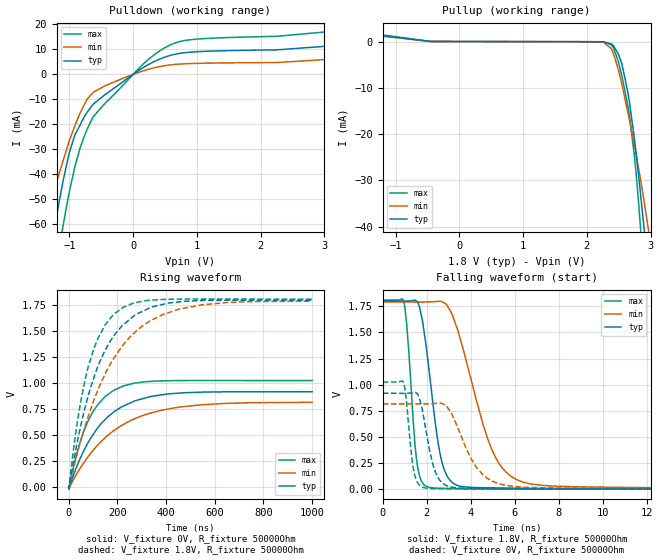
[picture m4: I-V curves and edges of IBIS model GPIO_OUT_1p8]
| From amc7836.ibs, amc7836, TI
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|   Model
[Model]   GPIO_OUT_1p8
Model_type   Output
Polarity   Non-Inverting
Vmeas = 0.9
Vref = 0
Cref = 1pF
Rref = 100000
|   typ   min   max
C_comp   2.855pF   2.622pF   2.914pF
[Voltage Range]   1.8   1.79   1.81
[Temperature Range]   27   125   -40
[Pullup Reference]   1.8   1.79   1.81
[Pulldown Reference]   0   0   0
[Power Clamp Reference]   1.8   1.79   1.81
[GND Clamp Reference]   0   0   0
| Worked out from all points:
|   slope of the pulldown table from 0 to 0.27 V, typ, clamps not added: 62.1 ohm
|   slope of the pullup table from 0 to 0.27 V, typ, clamps not added: 48 kohm
|   falling waveform, V_fixture 1.8V, R_fixture 50000Ohm: 20-80 % time 663ps typ, 1.47ns min, 359ps max; typ from 1.8 V to 0.004 V
|   rising waveform, V_fixture 0V, R_fixture 50000Ohm: 20-80 % time 161ns typ, 224ns min, 109ns max; typ from 0.002 V to 0.918 V
|   rising waveform, V_fixture 1.8V, R_fixture 50000Ohm: 20-80 % time 152ns typ, 207ns min, 104ns max; typ from 0.004 V to 1.8 V
|   falling waveform, V_fixture 0V, R_fixture 50000Ohm: 20-80 % time 539ps typ, 1.16ns min, 299ps max; typ from 0.919 V to 0.002 V
[Pulldown]
|   Voltage   I(typ)   I(min)   I(max)
-1.8V     -152.9mA   -105mA     -208.5mA
-1.422V   -90.58mA   -64.62mA   -123.9mA
-1.26V    -65.97mA   -48.83mA   -90.14mA
-1.199V   -56.75mA   -43.25mA   -77.47mA
-1.093V   -42.19mA   -34.3mA    -60.11mA
-995.4mV  -31.07mA   -26.33mA   -46.69mA
-833.4mV  -20.43mA   -15.7mA    -29.76mA
-644.4mV  -12.6mA    -7.83mA    -18mA
-444.6mV  -8.238mA   -4.696mA   -11.76mA
235.8mV   3.851mA    1.971mA    5.875mA
689.4mV   8.213mA    4.042mA    12.84mA
3.6V      12.34mA    6.871mA    18.33mA
[Pullup]
|   Voltage   I(typ)   I(min)   I(max)
-1.8V     2.219mA    2.026mA    2.51mA
-444.6mV  9.239uA    7.553uA    11.63uA
2.174V    -47.3uA    -58.31uA   -57.84uA
2.38V     -479.6uA   -1.489mA   -677.7uA
2.423V    -1.018mA   -2.833mA   -1.574mA
2.542V    -4.518mA   -8.772mA   -6.951mA
2.644V    -11.07mA   -15.39mA   -14mA
2.747V    -21.1mA    -22.53mA   -24.86mA
2.817V    -29.62mA   -27.82mA   -35.76mA
2.887V    -38.98mA   -33.59mA   -48.82mA
3.044V    -61.72mA   -47.7mA    -81.16mA
3.6V      -152.4mA   -105.9mA   -205.5mA
[Ramp]
R_load = 50000
|   typ   min   max
dV/dt_r   0.549882/1.61466e-07   0.488189/2.23683e-07   0.614755/1.08787e-07
dV/dt_f   1.07784/6.62535e-10   1.07057/1.46971e-09   1.08424/3.58989e-10
[Falling Waveform]
V_fixture = 1.8V
V_fixture_min = 1.79V
V_fixture_max = 1.81V
R_fixture = 50000Ohm
C_fixture = 0F
|   Time   V(typ)   V(min)   V(max)
0s        1.8V       1.791V     1.81V
950.4ps   1.8V       1.791V     1.798V
1.492ns   1.806V     1.791V     365mV
1.728ns   1.686V     1.791V     93.52mV
2.696ns   254.3mV    1.795V     9.896mV
3.737ns   23.69mV    1.277V     6.401mV
4.761ns   14.97mV    488.1mV    5.067mV
5.833ns   11.59mV    124.2mV    4.365mV
13.01ns   4.998mV    15.12mV    3.002mV
1us       3.902mV    6.729mV    2.919mV
[Rising Waveform]
V_fixture = 0V
V_fixture_min = 0V
V_fixture_max = 0V
R_fixture = 50000Ohm
C_fixture = 0F
|   Time   V(typ)   V(min)   V(max)
0s        1.97mV     3.048mV    1.633mV
771.6ps   -4.749mV   3.423mV    -19.59mV
23.52ns   140.4mV    88.54mV    233.3mV
45.68ns   268.2mV    176.6mV    424mV
92.98ns   481.1mV    333.2mV    698.2mV
149.5ns   651mV      475.5mV    872mV
224.4ns   780.5mV    603.8mV    974.5mV
340.3ns   874.8mV    715.9mV    1.018V
451.9ns   905mV      769.8mV    1.026V
1us       918.4mV    816.7mV    1.026V
[Rising Waveform]
V_fixture = 1.8V
V_fixture_min = 1.79V
V_fixture_max = 1.81V
R_fixture = 50000Ohm
C_fixture = 0F
|   Time   V(typ)   V(min)   V(max)
0s        3.902mV    6.729mV    2.919mV
771.6ps   -3.09mV    7.066mV    -16.2mV
39.91ns   488.3mV    363mV      691.7mV
77.83ns   861.2mV    664.4mV    1.137V
121.1ns   1.172V     941.9mV    1.437V
183.1ns   1.449V     1.234V     1.661V
304.3ns   1.694V     1.555V     1.791V
451.9ns   1.783V     1.713V     1.81V
647.3ns   1.8V       1.777V     1.811V
1us       1.8V       1.791V     1.81V
[Falling Waveform]
|Gnd
V_fixture = 0V
V_fixture_min = 0V
V_fixture_max = 0V
R_fixture = 50000Ohm
C_fixture = 0F
|   Time   V(typ)   V(min)   V(max)
0s        918.5mV    817mV      1.026V
950.4ps   918.1mV    816.8mV    1.018V
1.336ns   923.3mV    816.7mV    271.4mV
1.625ns   891.7mV    816.7mV    50.89mV
2.489ns   120.4mV    822.4mV    5.965mV
3.737ns   10.4mV     418.2mV    3.729mV
4.547ns   7.948mV    139.7mV    3.026mV
5.611ns   6.531mV    38.05mV    2.6mV
15.9ns    2.422mV    5.67mV     1.627mV
1us       1.97mV     3.048mV    1.633mV
